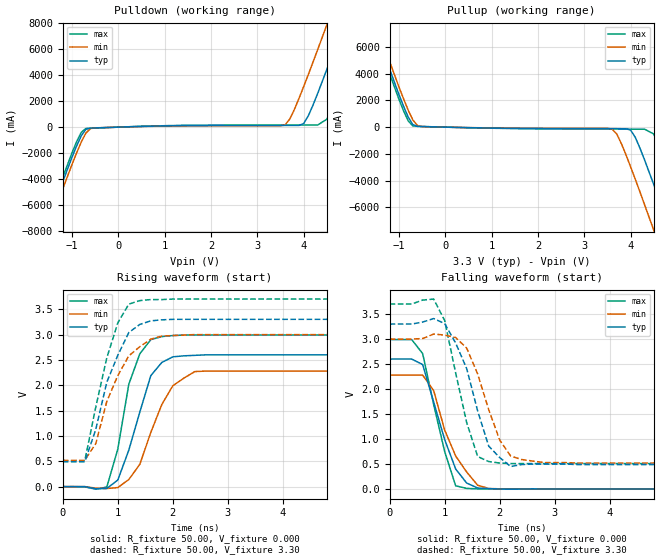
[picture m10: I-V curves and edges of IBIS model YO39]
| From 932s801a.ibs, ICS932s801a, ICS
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|   Model YO39
[Model]   YO39
Model_type   Output
Polarity   Non-Inverting
C_comp   2.0pF   1.5pF   2.5pF
[Temperature Range]   27.00   70.00   0.000
[Voltage Range]   3.30V   3.00V   3.70V
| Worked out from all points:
|   slope of the pulldown table from 0 to 0.495 V, typ, clamps not added: 8.8 ohm
|   slope of the pullup table from 0 to 0.495 V, typ, clamps not added: 12.8 ohm
|   rising waveform, R_fixture 50.00, V_fixture 0.000: 20-80 % time 437ps typ, 505ps min, 362ps max; typ from 0 V to 2.6 V
|   rising waveform, R_fixture 50.00, V_fixture 3.30: 20-80 % time 490ps typ, 521ps min, 431ps max; typ from 0.49 V to 3.3 V
|   falling waveform, R_fixture 50.00, V_fixture 0.000: 20-80 % time 450ps typ, 491ps min, 382ps max; typ from 2.6 V to 0 V
|   falling waveform, R_fixture 50.00, V_fixture 3.30: 20-80 % time 474ps typ, 467ps min, 395ps max; typ from 3.3 V to 0.49 V
[Pulldown]
| voltage   I(typ)   I(min)   I(max)
-3.3V     -24.7A     -25.47A    -24.37A
-1.7V     -8.96A     -9.5A      -8.61A
-1.5V     -7.02A     -7.57A     -6.67A
-900mV    -1.44A     -1.97A     -1.11A
-700mV    -160mA     -450mA     -100mA
3.6V      130mA      180mA      160mA
4V        280mA      3.13A      160mA
4.3V      2.58A      5.95A      160mA
4.5V      4.45A      7.88A      610mA
4.9V      8.31A      11.78A     4.11A
5.3V      12.23A     15.71A     7.98A
6.6V      25.12A     28.62A     20.83A
[Pullup]
| voltage   I(typ)   I(min)   I(max)
-3.3V     24.84A     25.38A     24.51A
-1.7V     9.1A       9.67A      8.75A
-1.5V     7.16A      7.73A      6.81A
-900mV    1.56A      2.12A      1.22A
-700mV    190mA      540mA      95.79mA
3.6V      -110mA     -140mA     -140mA
4V        -220mA     -2.96A     -150mA
4.3V      -2.43A     -5.78A     -150mA
4.5V      -4.29A     -7.7A      -510mA
4.9V      -8.15A     -11.6A     -3.98A
5.3V      -12.07A    -15.54A    -7.84A
6.6V      -24.97A    -28.46A    -20.7A
[Ramp]
| variable   typ   min   max
dV/dt_r   1.56/0.35n   1.37/0.48n   1.80/0.30n
dV/dt_f   1.68/0.41n   1.49/0.45n   1.91/0.31n
R_load = 50.00
[Rising Waveform]
R_fixture = 50.00
V_fixture = 0.000
V_fixture_min = 0.000
V_fixture_max = 0.000
| time   V(typ)   V(min)   V(max)
0s        180uV      0V         250uV
800ps     -36.04mV   -36.18mV   -8.17mV
1ns       130mV      -18.73mV   740mV
1.2ns     720mV      140mV      2.02V
1.4ns     1.47V      440mV      2.62V
1.6ns     2.19V      1.07V      2.9V
1.8ns     2.45V      1.62V      2.96V
2ns       2.56V      1.99V      2.98V
2.4ns     2.59V      2.27V      2.99V
10ns      2.6V       2.28V      2.99V
[Rising Waveform]
R_fixture = 50.00
V_fixture = 3.30
V_fixture_min = 3.00
V_fixture_max = 3.70
| time   V(typ)   V(min)   V(max)
0s        490mV      520mV      510mV
400ps     490mV      520mV      510mV
600ps     1.13V      850mV      1.57V
800ps     2.06V      1.68V      2.54V
1ns       2.59V      2.19V      3.23V
1.2ns     3.04V      2.58V      3.6V
1.4ns     3.2V       2.76V      3.67V
1.8ns     3.29V      2.97V      3.69V
2.4ns     3.3V       3V         3.7V
10ns      3.3V       3V         3.7V
[Falling Waveform]
R_fixture = 50.00
V_fixture = 0.000
V_fixture_min = 0.000
V_fixture_max = 0.000
| time   V(typ)   V(min)   V(max)
0s        2.6V       2.28V      2.99V
400ps     2.6V       2.28V      2.99V
600ps     2.49V      2.28V      2.71V
800ps     1.74V      1.97V      1.69V
1ns       990mV      1.18V      750mV
1.2ns     400mV      660mV      64.44mV
1.4ns     120mV      340mV      13.08mV
1.6ns     20.08mV    75.33mV    3.34mV
1.8ns     7.99mV     11.27mV    2.51mV
10ns      -15.58uV   -5.2uV     -3.88uV
[Falling Waveform]
R_fixture = 50.00
V_fixture = 3.30
V_fixture_min = 3.00
V_fixture_max = 3.70
| time   V(typ)   V(min)   V(max)
0s        3.3V       3V         3.7V
800ps     3.41V      3.1V       3.8V
1ns       3.31V      3.08V      3.37V
1.4ns     2.41V      2.82V      1.33V
1.6ns     1.56V      2.3V       650mV
1.8ns     860mV      1.59V      550mV
2ns       630mV      980mV      520mV
2.2ns     450mV      660mV      510mV
2.8ns     500mV      530mV      510mV
10ns      490mV      520mV      510mV
